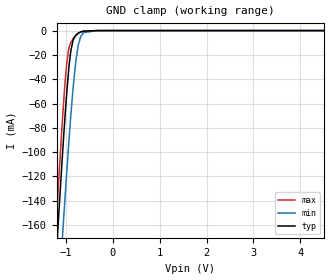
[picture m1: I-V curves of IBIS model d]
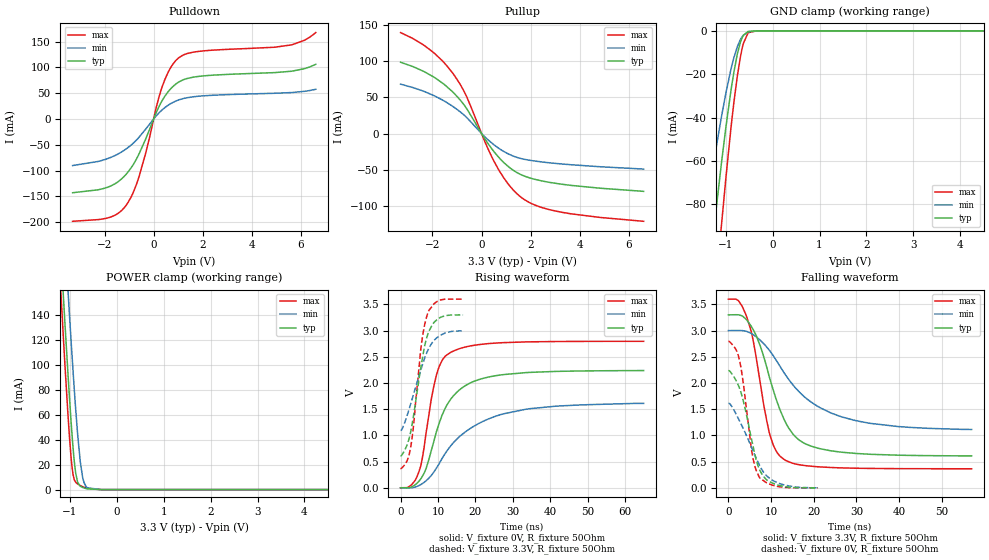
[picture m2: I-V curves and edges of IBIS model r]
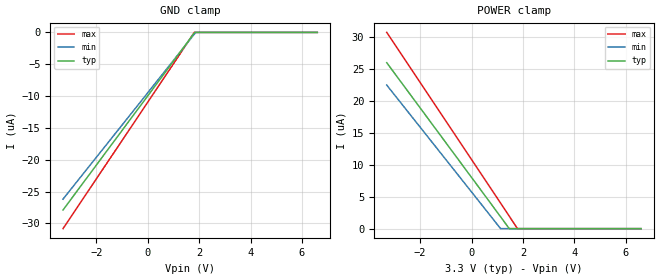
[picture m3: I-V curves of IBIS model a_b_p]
|Texas Instruments Incorporated
| 3.3-V-Supply Full-Duplex RS-485 with 16kV IEC61000-4-2 Contact Discharge
| ESD Protection
| Marketing part#   Digital Voltage Range   Package-type   #pins
| SN65HVD1474DGK   3.0V-3.6V   VSSOP   8
| SN65HVD1474DGKR   3.0V-3.6V   VSSOP   8
| SN65HVD1474D   3.0V-3.6V   SOIC   8
| SN65HVD1474DR   3.0V-3.6V   SOIC   8
[IBIS Ver]   4.1
[File name]   sn65hvd1474.ibs
[File Rev]   1.0
[Date]   6/26/2014
[Source]
| Texas Instruments Incorporated.
| Analog-eLab Design Center, HPA
| 12500 TI Blvd
| Dallas, TX -75243
[Notes]   Revision History:
| Rev 1.0: 6/26/2014
| - Relative part of SN65HVD74
| - Model generated from simulations in TISPICE
| - Model matched to SPICE simulation
| - C_comp although listed in numerical order of value are
|   obtained from varying PVT conditions. For PVT conditions for
|   each specific value refer the buffer description under
|   respective [Model]. IBIS model user is responsible for using
|   appropriate C_comp to simulate for Signal Integrity.
|* EXCEPTION:   *
|* - For model d, there is leakage current in the GND   *
|*   clamp I-V Table because of the pullup on pad.   *
|* - For models a_b_p and a_b_n, there is leakage current in the   *
|*   POWER clamp and GND clamp I-V Table because of the resistor   *
|*   network connected to pad.   *
[Disclaimer]
| This model is designed as an aid for customers of Texas Instruments.
| TI and its licensors and suppliers make no warranties, either expressed
| or implied, with respect to this  model, including the warranties of
| merchantability or fitness for a particular purpose. The model is
| provided solely on an "as is" basis. The entire risk as to its quality
| and performance is with the customer.
[Copyright]
(C) Copyright 2014 Texas Instruments Incorporated.All rights reserved.
|   SN65HVD1474DGK
[Component]   SN65HVD1474DGK
[Manufacturer]   TI
[Package]   |8 VSSOP  -  DGK package
|   typ   min   max
R_pkg   0.2   0.16   0.24
L_pkg   1.5nH   1.2nH   1.8nH
C_pkg   0.4pF   0.32pF   0.48pF
[Pin]  signal_name   model_name   R_pin   L_pin   C_pin
1   VCC   power   NA   NA   NA
2   R   r   NA   NA   NA
3   D   d   NA   NA   NA
4   GND   gnd   NA   NA   NA
5   Y   y_z_p   NA   NA   NA
6   Z   y_z_n   NA   NA   NA
7   B   a_b_n   NA   NA   NA
8   A   a_b_p   NA   NA   NA
[Diff_pin]   inv_pin   vdiff   tdelay_typ   tdelay_min   tdelay_max
5   6   0V   NA   NA   NA
8   7   0.2V   NA   NA   NA
|   SN65HVD1474D
[Component]   SN65HVD1474D
[Manufacturer]   TI
[Package]   |8 SOIC   -  D package
|   typ   min   max
R_pkg   0.2   0.16   0.24
L_pkg   1.5nH   1.2nH   1.8nH
C_pkg   0.4pF   0.32pF   0.48pF
[Pin]  signal_name   model_name   R_pin   L_pin   C_pin
1   VCC   power   NA   NA   NA
2   R   r   NA   NA   NA
3   D   d   NA   NA   NA
4   GND   gnd   NA   NA   NA
5   Y   y_z_p   NA   NA   NA
6   Z   y_z_n   NA   NA   NA
7   B   a_b_n   NA   NA   NA
8   A   a_b_p   NA   NA   NA
[Diff_pin]   inv_pin   vdiff   tdelay_typ   tdelay_min   tdelay_max
5   6   0V   NA   NA   NA
8   7   0.2V   NA   NA   NA
| Models and submodels in the file (6): d (Input), r (3-state), a_b_p (Input), a_b_n (Input), y_z_p (Output), y_z_n (Output)
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|   d Model
[Model]   d
Model_type   Input
Vinl = 0.8
Vinh = 2
|   typ   min   max
|   (nom PVT)   (fast PVT)   (slow PVT)
C_comp   8.114e-13   7.750e-13   8.695e-13
| Where nom  PVT is Nominal Process, 3.3V, 27C
|   Fast PVT is Strong Process,  3.6V, -40C
|   Slow PVT is Weak Process,   3V, 150C
[Voltage Range]   3.3   3   3.6
|Junction Temperature
[Temperature Range]   27   150   -40
[Power Clamp Reference]   3.3   3   3.6
[GND Clamp Reference]   0   0   0
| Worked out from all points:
|   GND clamp passes 1 mA (typ) near -0.67 V on its own axis
[GND Clamp]
|   Voltage   I(typ)   I(min)   I(max)
-3.3V     -1.706A    -1.709A    -1.74A
-1.33V    -268.5mA   -332.2mA   -244.5mA
-1.176V   -166.3mA   -233.3mA   -138.2mA
-1.064V   -96.82mA   -164.4mA   -67.68mA
-980.1mV  -50.33mA   -115.2mA   -26.33mA
-945.6mV  -34.42mA   -96.08mA   -16.53mA
-891mV    -15.86mA   -67.76mA   -9.449mA
-789mV    -3.689mA   -25.45mA   -4.166mA
-735mV    -2.045mA   -11.84mA   -2.349mA
-686.4mV  -1.145mA   -5.17mA    -1.213mA
-330mV    -2.214uA   -10.64uA   -3.071uA
6.6V      0A         0A         0A
[POWER Clamp]
|   Voltage   I(typ)   I(min)   I(max)
-3.3V     0A         0A         0A
0V        0A         0A         0A
6.6V      0A         0A         0A
|   r Model
[Model]   r
Model_type   3-state
Polarity   Non-Inverting
Vmeas = 1.65
Vref = 0
Cref = 2pF
Rref = 70
|   typ   min   max
|   (nom PVT)   (fast PVT)   (slow PVT)
C_comp   2.588e-12   2.046e-12   2.817e-12
| Where nom  PVT is Nominal Process, 3.3V, 27C
|   Fast PVT is Strong Process,  3.6V, -40C
|   Slow PVT is Weak Process,   3V, 150C
[Voltage Range]   3.3   3   3.6
|Junction Temperature
[Temperature Range]   27   150   -40
[Pullup Reference]   3.3   3   3.6
[Pulldown Reference]   0   0   0
[Power Clamp Reference]   3.3   3   3.6
[GND Clamp Reference]   0   0   0
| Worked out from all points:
|   slope of the pulldown table from 0 to 0.495 V, typ, clamps not added: 10.6 ohm
|   slope of the pullup table from 0 to 0.495 V, typ, clamps not added: 20.2 ohm
|   GND clamp passes 1 mA (typ) near -0.56 V on its own axis
|   POWER clamp passes 1 mA (typ) near -0.67 V on its own axis
|   falling waveform, V_fixture 3.3V, R_fixture 50Ohm: 20-80 % time 6.87ns typ, 12.8ns min, 4.29ns max; typ from 3.3 V to 0.61 V
|   rising waveform, V_fixture 0V, R_fixture 50Ohm: 20-80 % time 7.42ns typ, 13.6ns min, 4.14ns max; typ from 0 V to 2.24 V
|   rising waveform, V_fixture 3.3V, R_fixture 50Ohm: 20-80 % time 3.7ns typ, 5.09ns min, 2.84ns max; typ from 0.607 V to 3.3 V
|   falling waveform, V_fixture 0V, R_fixture 50Ohm: 20-80 % time 3.78ns typ, 5.51ns min, 2.72ns max; typ from 2.24 V to 0 V
[Pulldown]
|   Voltage   I(typ)   I(min)   I(max)
-3.3V     -142.9mA   -90.24mA   -198.2mA
-1.752V   -129.9mA   -74.58mA   -190mA
-1.313V   -116.4mA   -64.07mA   -177.8mA
-1.05V    -103.1mA   -55.56mA   -162.3mA
-592.8mV  -67.39mA   -35.2mA    -111.3mA
114mV     13.41mA    6.499mA    24.02mA
346.5mV   35.66mA    17.65mA    62.34mA
663mV     57.01mA    28.87mA    97.12mA
1.042V    72.13mA    37.29mA    119.3mA
1.821V    82.45mA    44.04mA    130.9mA
5.581V    92.36mA    51.13mA    143.3mA
6.6V      105.9mA    57.57mA    167.4mA
[GND Clamp]
|   Voltage   I(typ)   I(min)   I(max)
-3.3V     -803.1mA   -470.3mA   -1.084A
-1.502V   -143.6mA   -96.84mA   -192.8mA
-1.356V   -113mA     -75.22mA   -155.4mA
-1.206V   -82.91mA   -54.43mA   -117.7mA
-1.093V   -61.63mA   -40.07mA   -90.45mA
-895.2mV  -28.72mA   -18.5mA    -46.5mA
-825mV    -19.08mA   -12.43mA   -33.02mA
-751.2mV  -10.69mA   -7.305mA   -20.87mA
-686.4mV  -5.303mA   -4.059mA   -12.14mA
-625.2mV  -2.182mA   -2.075mA   -5.962mA
-520.8mV  -269.2uA   -497.1uA   -854.5uA
6.6V      0A         0A         0A
[Pullup]
|   Voltage   I(typ)   I(min)   I(max)
-3.3V     98.28mA    68.06mA    139.2mA
-2.782V   92.06mA    63.21mA    130.7mA
-1.98V    78.53mA    52.86mA    112.3mA
-1.175V   57.31mA    37.47mA    83.24mA
-603.9mV  34.27mA    22.05mA    50.6mA
161.7mV   -8.749mA   -5.451mA   -13.35mA
656.7mV   -31.16mA   -19.34mA   -47.56mA
1.128V    -46.6mA    -28.71mA   -71.43mA
1.593V    -56.5mA    -34.39mA   -87.39mA
2.185V    -63.25mA   -37.99mA   -98.76mA
3.231V    -69.71mA   -41.87mA   -108.3mA
6.6V      -79.71mA   -48.99mA   -121mA
[POWER Clamp]
|   Voltage   I(typ)   I(min)   I(max)
-3.3V     1.726A     1.762A     1.723A
-1.273V   245.9mA    312.1mA    214.3mA
-1.14V    156.3mA    223.7mA    123.1mA
-1.036V   90.42mA    157.4mA    57.82mA
-953.7mV  44.13mA    107.5mA    18.25mA
-910.8mV  24.82mA    83.2mA     8.67mA
-874.5mV  13.09mA    63.93mA    5.84mA
-777mV    2.686mA    22.24mA    3.242mA
-729mV    1.724mA    10.13mA    2.356mA
-627mV    626uA      1.45mA     889.8uA
-330mV    1.075uA    8.852uA    372.3nA
6.6V      0A         0A         0A
[Ramp]
R_load = 50
|   typ   min   max
dV/dt_r   1.34256/7.38446e-09   0.966209/1.35443e-08  1.67737/4.13854e-09
dV/dt_f   1.61569/6.86378e-09   1.1409/1.30249e-08   1.94163/4.29016e-09
[Falling Waveform]
V_fixture = 3.3V
V_fixture_min = 3V
V_fixture_max = 3.6V
R_fixture = 50Ohm
|   Time   V(typ)   V(min)   V(max)
0s        3.3V       3V         3.6V
2.315ns   3.301V     3.002V     3.573V
4.31ns    3.2V       2.983V     3.255V
5.83ns    3.014V     2.921V     2.797V
9.725ns   2.076V     2.611V     1.009V
11.41ns   1.639V     2.407V     672.8mV
13ns      1.313V     2.2V       546mV
17.65ns   856.3mV    1.748V     428.5mV
26.75ns   678.5mV    1.349V     380.5mV
57ns      610.1mV    1.114V     364.2mV
[Rising Waveform]
V_fixture = 0V
V_fixture_min = 0V
V_fixture_max = 0V
R_fixture = 50Ohm
|   Time   V(typ)   V(min)   V(max)
0s        1.908nV    301.7nV    275.6pV
2.705ns   9.001mV    -576.3uV   43.23mV
4.785ns   113.4mV    36.79mV    278.6mV
6.78ns    359mV      130.5mV    1.022V
9.56ns    1.06V      370.2mV    2.14V
11.31ns   1.42V      582.8mV    2.453V
13.48ns   1.698V     805.8mV    2.588V
18.92ns   2.01V      1.145V     2.711V
27.45ns   2.16V      1.41V      2.77V
64.99ns   2.238V     1.61V      2.796V
[Rising Waveform]
V_fixture = 3.3V
V_fixture_min = 3V
V_fixture_max = 3.6V
R_fixture = 50Ohm
|   Time   V(typ)   V(min)   V(max)
0s        606.8mV    1.095V     363.9mV
1.755ns   820.5mV    1.377V     515.1mV
2.79ns    1.094V     1.618V     806.8mV
3.505ns   1.387V     1.789V     1.211V
5.405ns   2.288V     2.243V     2.64V
6.21ns    2.616V     2.423V     3.027V
7.31ns    2.934V     2.624V     3.337V
8.915ns   3.153V     2.81V      3.509V
10.64ns   3.251V     2.911V     3.585V
16.72ns   3.299V     2.998V     3.6V
[Falling Waveform]
V_fixture = 0V
V_fixture_min = 0V
V_fixture_max = 0V
R_fixture = 50Ohm
|   Time   V(typ)   V(min)   V(max)
0s        2.238V     1.614V     2.796V
1.81ns    2.044V     1.405V     2.632V
2.65ns    1.888V     1.268V     2.412V
3.525ns   1.645V     1.121V     1.973V
5.4ns     933.5mV    776.2mV    722.4mV
6.18ns    646.8mV    624.7mV    416.7mV
7.365ns   334.6mV    418.9mV    188.7mV
8.985ns   151.7mV    226.7mV    94.37mV
11.72ns   50.31mV    90.48mV    23.57mV
21ns      253.8uV    1.73mV     115.9uV
|   a_b Model
[Model]   a_b_p
Model_type   Input
Vinl = 0.8
Vinh = 2
|   typ   min   max
|   (nom PVT)   (fast PVT)   (slow PVT)
C_comp   3.624e-12   3.555e-12   3.721e-12
| Where nom  PVT is Nominal Process, 3.3V, 27C
|   Fast PVT is Strong Process,  3.6V, -40C
|   Slow PVT is Weak Process,   3V, 150C
[Voltage Range]   3.3   3   3.6
|Junction Temperature
[Temperature Range]   27   150   -40
[Power Clamp Reference]   3.3   3   3.6
[GND Clamp Reference]   0   0   0
[GND Clamp]
|   Voltage   I(typ)   I(min)   I(max)
-3.3V     -27.91uA   -26.2uA    -30.84uA
1.808V    -113nA     -299.4nA   -15.76nA
1.872V    0A         0A         0A
6.6V      0A         0A         0A
[POWER Clamp]
|   Voltage   I(typ)   I(min)   I(max)
-3.3V     25.96uA    22.46uA    30.7uA
1.131V    1.86uA     8.519nA    4.006uA
1.468V    13.45nA    0A         1.955uA
1.787V    0A         0A         13.55nA
6.6V      0A         0A         0A
